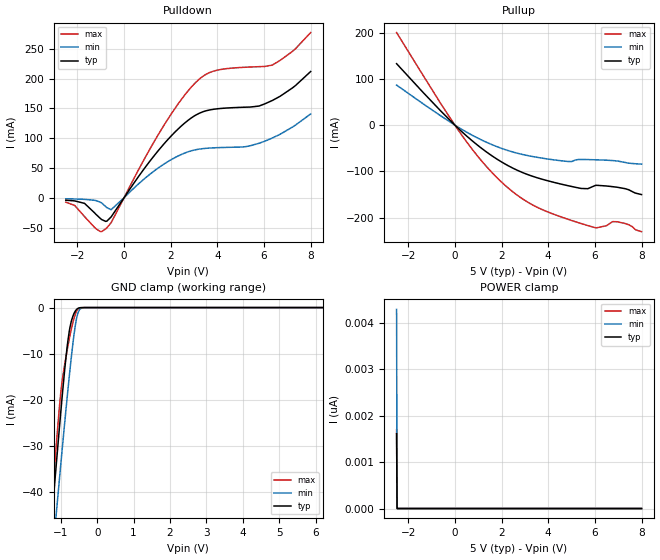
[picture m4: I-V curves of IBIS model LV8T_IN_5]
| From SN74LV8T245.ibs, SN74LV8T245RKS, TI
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[Model]   LV8T_IN_5
Model_type   Input
Vinl = 0.8
Vinh = 2
|   typ   min   max
C_comp   4.5pF   4.4pF   4.7pF
[Voltage Range]   5   4.5   5.5
[Temperature Range]   25   125   -40
[Power Clamp Reference]   5   4.5   5.5
[GND Clamp Reference]   0   0   0
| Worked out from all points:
|   slope of the pulldown table from 0 to 0.75 V, typ, clamps not added: 17.6 ohm
|   slope of the pullup table from 0 to 0.75 V, typ, clamps not added: 22 ohm
|   GND clamp passes 1 mA (typ) near -0.62 V on its own axis
[Pulldown]
|   Voltage   I(typ)   I(min)   I(max)
-2.5V     -4.172mA   -1.772mA   -7.441mA
-2.122V   -5.347mA   -2.105mA   -12.9mA
-1.702V   -9.4mA     -2.721mA   -31.36mA
-1.009V   -35.09mA   -7.698mA   -56.94mA
-788.5mV  -39.73mA   -14.85mA   -52.23mA
-557.5mV  -32.38mA   -20.14mA   -42.06mA
1.605V    85.59mA    53.79mA    115mA
3.075V    138.8mA    80.61mA    193.8mA
3.958V    149.1mA    83.96mA    213.8mA
5.28V     152.1mA    86.22mA    219.2mA
6.351V    163.2mA    100.1mA    222.7mA
8V        211.9mA    140.7mA    277.3mA
[GND Clamp]
|   Voltage   I(typ)   I(min)   I(max)
-2.5V     -170.7mA   -168.9mA   -187.4mA
-1.282V   -49.09mA   -58.54mA   -46.61mA
-1.24V    -45.04mA   -54.83mA   -42.02mA
-1.208V   -42.02mA   -52.06mA   -38.61mA
-1.125V   -34.05mA   -44.71mA   -29.82mA
-977.5mV  -20.62mA   -32.07mA   -16.86mA
-799mV    -6.847mA   -17.4mA    -8.124mA
-715mV    -3.091mA   -11.05mA   -4.817mA
-641.5mV  -1.357mA   -6.134mA   -2.454mA
-526mV    -161.3uA   -1.092mA   -287.1uA
-379mV    -1.459uA   -24.15uA   -792nA
8V        0A         0A         0A
[Pullup]
|   Voltage   I(typ)   I(min)   I(max)
-2.5V     133.2mA    86.83mA    200.6mA
-610mV    30.93mA    20.35mA    46.86mA
429.5mV   -20.16mA   -13.03mA   -31.05mA
1.406V    -59.92mA   -38.19mA   -92.51mA
2.341V    -89.31mA   -55.94mA   -138.5mA
3.517V    -113.7mA   -69.57mA   -177.5mA
4.84V     -131mA     -78.59mA   -203.7mA
5.197V    -134.8mA   -75.08mA   -209.6mA
5.7V      -137.5mA   -74.5mA    -217.5mA
6.068V    -130.3mA   -75.07mA   -222.2mA
6.971V    -134.5mA   -77.65mA   -209.3mA
8V        -150.3mA   -84.36mA   -230.6mA
[POWER Clamp]
|   Voltage   I(typ)   I(min)   I(max)
-2.5V     1.613nA    4.292nA    1.698nA
-2.479V   0A         0A         0A
-2.469V   0A         0A         0A
8V        0A         0A         0A
